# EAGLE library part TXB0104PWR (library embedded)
Level Translator Voltage Levels 4-Bit Bi-directional V-Level Translator Hook-Up Guide: TXB0104 Level Shifter Hookup Guide
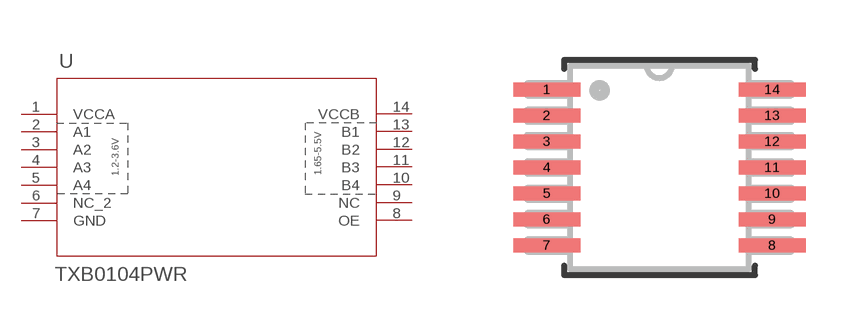
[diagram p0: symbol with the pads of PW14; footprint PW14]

Designator prefix U

## TXB0104PWR (DATASHEET: http://www.ti.com/lit/ds/symlink/txb0104.pdf; DESCR: Translation - Voltage Levels 4-Bit Bi-directional V-Level Translator; FARNELL_NO: 1607891; MF: Texas Instruments; MF_PN: TXB0104PWR; MOUSER_NO: 595-TXB0104PWR; PACKAGE: TSSOP-14; PURCHASE: https://de.farnell.com/texas-instruments/txb0104pwr/ic-sm-logik-translator/dp/1607891; UNIT_PRICE: 1.11)  [PW14]
1  VCCA  pwr
2  A1
3  A2
4  A3
5  A4
6  NC_2  nc
7  GND  pwr
8  OE
9  NC  nc
10  B4
11  B3
12  B2
13  B1
14  VCCB  pwr

## Footprint PW14 (pad centres in mm)
smd 1.676 x 0.356: 1 -2.819,1.95; 2 -2.819,1.3; 3 -2.819,0.65; 4 -2.819,0; 5 -2.819,-0.65; 6 -2.819,-1.3; 7 -2.819,-1.95; 8 2.819,-1.95; 9 2.819,-1.3; 10 2.819,-0.65; 11 2.819,0; 12 2.819,0.65; 13 2.819,1.3; 14 2.819,1.95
